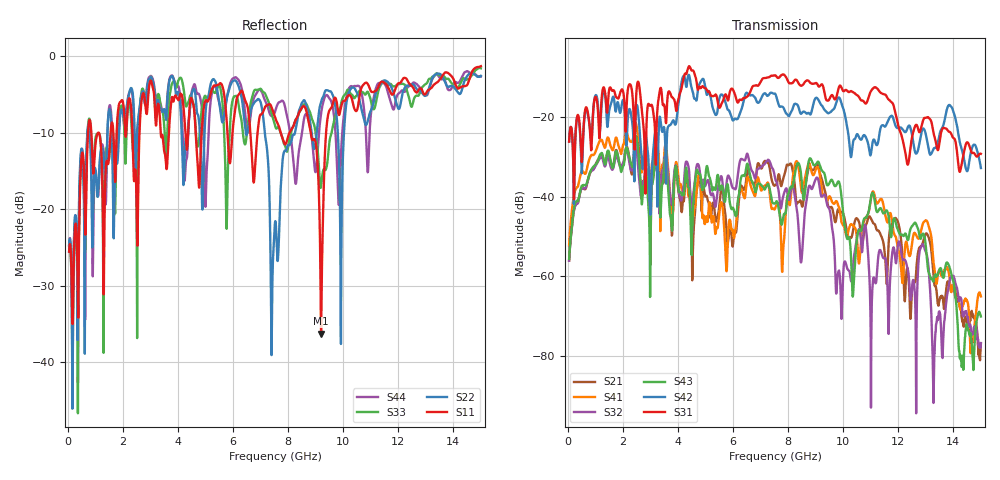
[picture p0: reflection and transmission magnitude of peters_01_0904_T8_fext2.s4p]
# MHZ S RI R 50.00
! FREQ  S11  S12  S13  S14
!  S21  S22  S23  S24
!  S31  S32  S33  S34
!  S41  S42  S43  S44
!  REAL  IMAG  REAL  IMAG  REAL  IMAG  REAL  IMAG
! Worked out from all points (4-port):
!   1496 points, 50 MHz to 15 GHz, reference 50 ohm
!   strongest paths, dB at 50 MHz, 3.79 GHz, 7.53 GHz, 11.27 GHz, 15 GHz:
!     S31: -26.2, -15.0, -9.5, -13.1, -29.2
!     S42: -26.1, -21.3, -14.2, -26.3, -32.8
!     S43: -55.6, -48.5, -41.7, -43.6, -70.0
!     S32: -56.0, -41.9, -35.4, -55.3, -76.7
!     S41: -52.2, -44.0, -42.9, -41.5, -65.0
!     S21: -56.0, -49.6, -37.1, -48.5, -76.8
!   lowest |S11| = -36.3 dB at 9.2 GHz (marker M1), VSWR 1.03, Z = 50.4 - j1.5 ohm
!   |S11| at or under -10 dB: start of sweep to 735.4 MHz; 1.133 GHz to 1.553 GHz (420.1 MHz wide, 31.3 % of centre); 8.823 GHz to 9.378 GHz (555.9 MHz wide, 6.11 % of centre)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
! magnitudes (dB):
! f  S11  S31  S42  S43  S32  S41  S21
! 50 MHz  -25.5  -26.2  -26.1  -55.6  -56.0  -52.2  -56.0
! 2.47 GHz  -15.4  -17.0  -18.7  -24.8  -26.6  -21.5  -25.4
! 5.75 GHz  -7.4  -14.5  -16.9  -38.7  -37.6  -57.7  -46.9
! 7.43 GHz  -6.9  -9.6  -14.0  -41.5  -32.9  -43.0  -36.3
! 9.2 GHz  -36.3  -11.9  -17.0  -33.0  -39.8  -37.1  -35.1
! 10.36 GHz  -6.2  -13.8  -26.2  -64.6  -57.4  -47.3  -48.4
! 15 GHz  -1.3  -29.2  -32.8  -70.0  -76.7  -65.0  -76.8
